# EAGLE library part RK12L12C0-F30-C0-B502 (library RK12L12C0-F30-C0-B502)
Potentiometers 12MM Source: Datasheet
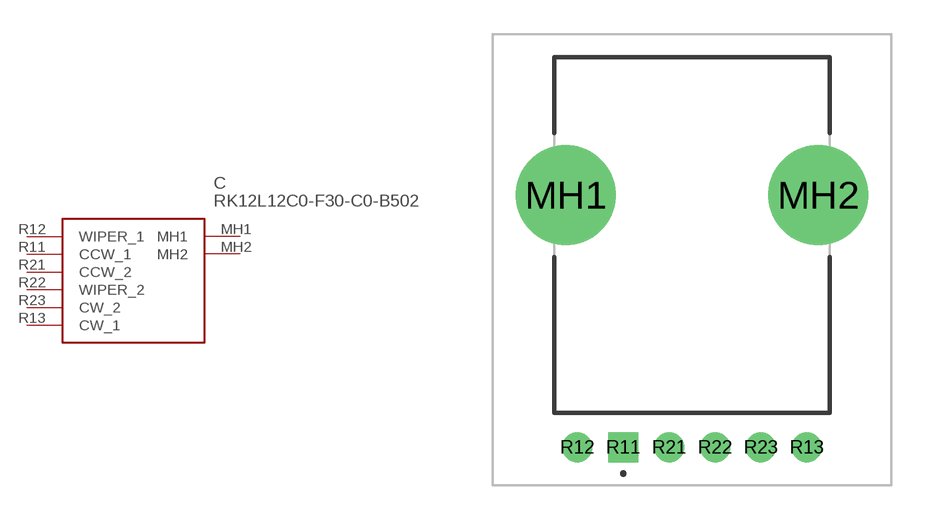
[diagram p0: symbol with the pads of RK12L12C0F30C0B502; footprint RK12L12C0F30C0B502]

Designator prefix C

## RK12L12C0-F30-C0-B502 (Description: Potentiometers 12MM; Height: 30mm; Manufacturer_Name: ALPS Electric; Manufacturer_Part_Number: RK12L12C0-F30-C0-B502)  [RK12L12C0F30C0B502]
MH1  MH1
MH2  MH2
R11  CCW_1
R12  WIPER_1
R13  CW_1
R21  CCW_2
R22  WIPER_2
R23  CW_2

## Footprint RK12L12C0F30C0B502 (pad centres in mm)
RK12L12C0-F30-C0-B502-1
drill 2.9 pad 4.35: MH1 -2.5,11; MH2 8.5,11
drill 0.8 pad 1.3 square: R11 0,0
drill 0.8 pad 1.3: R12 -2,0; R13 8,0; R21 2,0; R22 4,0; R23 6,0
